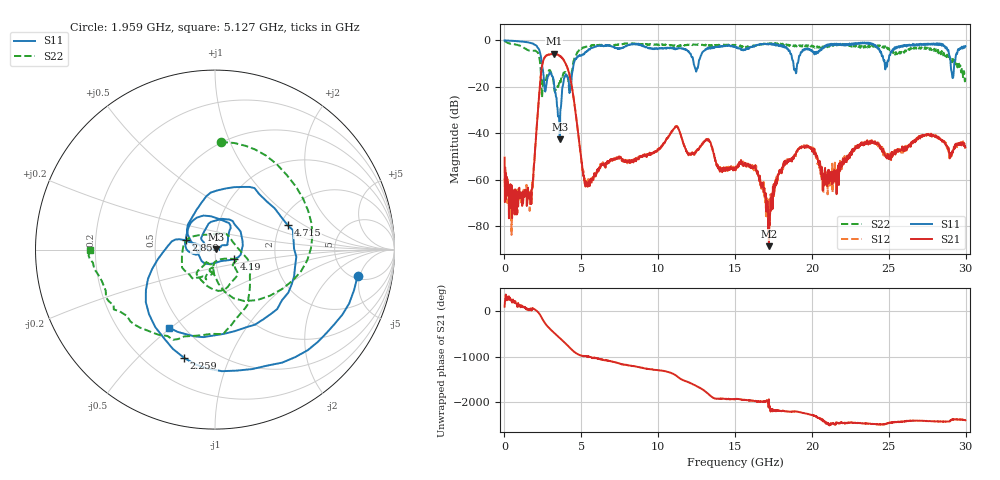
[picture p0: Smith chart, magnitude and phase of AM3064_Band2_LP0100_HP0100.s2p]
# Hz S DB R 50.0
!freq dBS11 angS11 dBS21 angS21 dBS12 angS12 dBS22 angS22
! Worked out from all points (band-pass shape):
!   1600 points, 10 MHz to 29.98 GHz, reference 50 ohm
!   highest |S21| = -5.74 dB at 3.215 GHz (marker M1); lowest = -88.6 dB at 17.2 GHz (marker M2)
!   |S21| within 3 dB of the highest: 2.525 GHz to 3.878 GHz (1.352 GHz wide, 42.2 % of centre)
!   lowest |S11| = -42.6 dB at 3.59 GHz (marker M3), VSWR 1.01, Z = 50.7 + j0.132 ohm
!   |S11| at or under -10 dB: 2.432 GHz to 4.506 GHz (2.075 GHz wide, 59.8 % of centre); 12.31 GHz to 12.62 GHz (311.2 MHz wide, 2.5 % of centre); 18.8 GHz to 19.05 GHz (252.5 MHz wide, 1.33 % of centre)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
!   |S22| runs from -24.6 to -0.3 dB; largest |S21 - S12| = 0.018
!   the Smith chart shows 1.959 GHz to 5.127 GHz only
!   S11 on the Smith chart (normalised r, x): 1.959 GHz: 5.50, -4.60; 2.259 GHz: 0.35, -0.69; 2.859 GHz: 0.71, +0.08; 4.19 GHz: 1.23, -0.13; 4.715 GHz: 2.20, +0.73; 5.127 GHz: 0.42, -0.49
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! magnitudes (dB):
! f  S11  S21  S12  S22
! 10 MHz  0.0  -50.5  -59.5  -0.3
! 1.603 GHz  -0.9  -66.2  -67.3  -4.4
! 1.959 GHz  -1.9  -50.4  -50.2  -4.4
! 2.259 GHz  -4.1  -23.3  -23.2  -7.3
! 2.859 GHz  -15.3  -6.2  -6.2  -13.6
! 3.215 GHz  -18.2  -5.7  -5.9  -19.6
! 3.59 GHz  -42.6  -6.5  -6.7  -17.0
! 4.19 GHz  -18.4  -13.7  -13.9  -20.0
! 4.715 GHz  -7.4  -35.9  -35.7  -5.4
! 5.015 GHz  -6.5  -52.9  -51.5  -3.7
! 5.127 GHz  -6.0  -58.2  -56.1  -3.1
! 10 GHz  -3.5  -47.0  -47.0  -1.8
! 11.2 GHz  -3.6  -37.1  -37.1  -2.4
! 15 GHz  -2.7  -55.0  -55.5  -2.0
! 16.34 GHz  -2.3  -55.0  -55.2  -2.4
! 17.2 GHz  -1.6  -88.6  -74.1  -1.6
! 18.19 GHz  -2.3  -53.9  -52.8  -1.9
! 19.99 GHz  -4.4  -46.6  -46.9  -2.2
! 20.87 GHz  -2.3  -59.2  -60.6  -3.0
! 23.23 GHz  -1.3  -45.1  -44.2  -2.7
! 25 GHz  -8.3  -50.4  -49.7  -3.3
! 29.98 GHz  -2.5  -46.0  -46.4  -15.8
